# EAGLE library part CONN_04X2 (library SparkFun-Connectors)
Multi connection point. Often used as Generic Header-pin footprint for 0.1 inch spaced/style header connections On any of the 0.1 inch spaced packages, you can populate with these: Break Away Headers - Straight (PRT-00116) Break Away Male Headers - Right Angle (PRT-00553) Female Headers (PRT-00115) Break Away Headers - Machine Pin (PRT-00117) Break Away Female Headers - Swiss Machine Pin (PRT-00743)
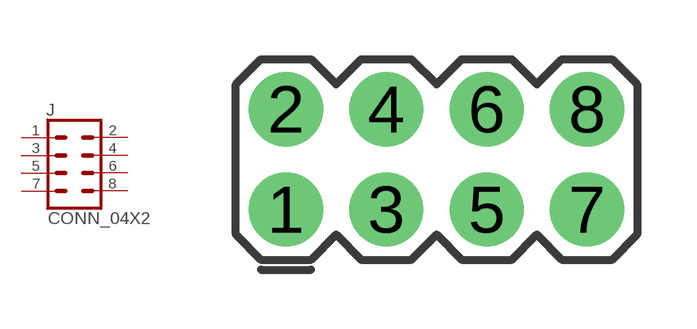
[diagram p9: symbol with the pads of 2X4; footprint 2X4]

Designator prefix J

## CONN_04X2  [2X4]
1  1  pas
2  2  pas
3  3  pas
4  4  pas
5  5  pas
6  6  pas
7  7  pas
8  8  pas

## Footprint 2X4 (pad centres in mm)
Plated Through Hole - 2x4 Specifications: Pin count:8 Pin pitch:0.1" Example device(s): CONN_04x2
drill 1.016 pad 1.88: 1 -3.81,-1.27; 2 -3.81,1.27; 3 -1.27,-1.27; 4 -1.27,1.27; 5 1.27,-1.27; 6 1.27,1.27; 7 3.81,-1.27; 8 3.81,1.27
